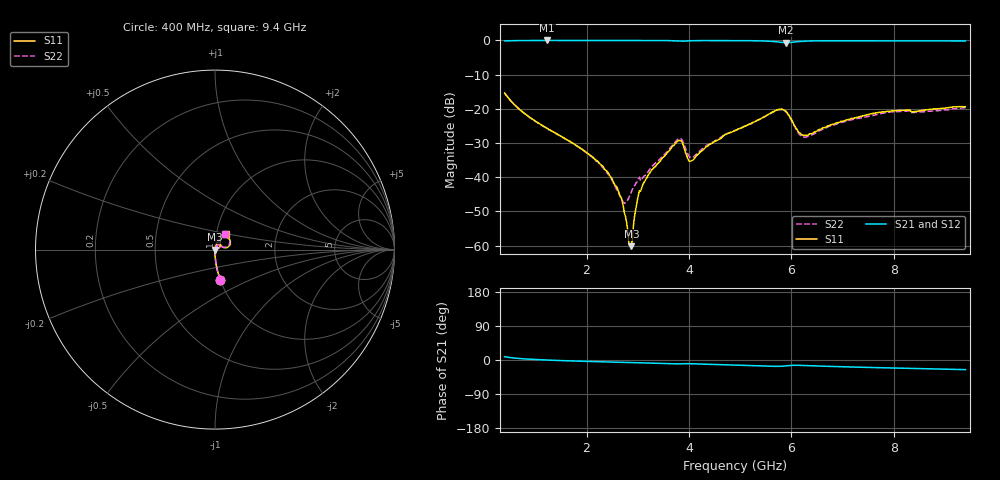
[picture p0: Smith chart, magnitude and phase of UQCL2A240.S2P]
! AVX Corporation
! Date:  10/27/06
! Part No:  UQCL2A240
! Description:  Ultra Low ESR Microwave capacitors
! Mounting Orientation:  Horizontal
# GHZ S DB R 50
! Freq  |S11|  S11 Ph  |S21|  S21 Ph  |S12|  S12 Ph  |S22|  S22 Ph
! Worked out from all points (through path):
!   401 points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, 400 MHz to 9.4 GHz, reference 50 ohm
!   highest |S21| = -0.02 dB at 1.233 GHz (marker M1); lowest = -0.7 dB at 5.89 GHz (marker M2)
!   group delay of S21, straight-line fit = 8.57 ps
!   lowest |S11| = -60.2 dB at 2.875 GHz (marker M3), VSWR 1.00, Z = 50.1 + j0.0469 ohm
!   |S11| at or under -10 dB: start of sweep to end of sweep
!   |S22| runs from -47.6 to -15.4 dB; largest |S21 - S12| = 0.0044
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0.4  -15.41 -80.3  -0.14 8.8  -0.14 8.7  -15.40 -80.1
1.233  -25.73 -88.5  -0.02 -0.2  -0.02 -0.3  -25.80 -87.0
1.908  -31.77 -90.1  -0.02 -3.3  -0.02 -3.3  -31.85 -85.4
2.268  -36.24 -89.6  -0.02 -4.6  -0.01 -4.7  -36.39 -79.5
2.538  -41.88 -86.8  -0.02 -5.6  -0.01 -5.7  -42.06 -66.4
2.65  -45.36 -80.5  -0.03 -6.0  -0.02 -6.1  -45.33 -48.3
2.74  -50.45 -76.4  -0.03 -6.4  -0.02 -6.4  -47.62 -15.5
2.83  -59.72 -40.5  -0.03 -6.7  -0.02 -6.7  -45.90 15.1
2.875  -60.18 28.6  -0.03 -6.8  -0.03 -6.9  -44.26 27.9
2.988  -47.11 88.2  -0.03 -7.2  -0.02 -7.3  -41.26 41.0
3.055  -44.09 78.8  -0.03 -7.4  -0.02 -7.5  -41.02 44.4
3.415  -35.72 74.3  -0.04 -8.7  -0.03 -8.9  -35.02 59.2
3.798  -29.31 50.2  -0.17 -10.3  -0.17 -10.4  -28.79 45.7
4.045  -35.26 50.7  -0.10 -9.9  -0.10 -10.0  -34.28 42.4
4.9  -26.35 69.5  -0.06 -13.2  -0.07 -13.3  -26.36 68.5
5.71  -20.37 45.8  -0.42 -16.8  -0.44 -16.8  -20.51 47.6
5.89  -20.68 21.9  -0.67 -15.4  -0.69 -15.4  -20.88 23.9
6.183  -27.24 22.6  -0.29 -14.2  -0.31 -14.0  -27.83 26.3
6.408  -27.25 48.2  -0.16 -15.3  -0.15 -15.2  -27.59 54.1
6.948  -23.88 61.4  -0.10 -17.7  -0.08 -17.7  -24.08 67.3
7.915  -20.70 58.1  -0.13 -20.9  -0.13 -21.0  -20.96 66.0
9.4  -19.40 53.8  -0.17 -25.4  -0.18 -25.5  -19.62 58.4
